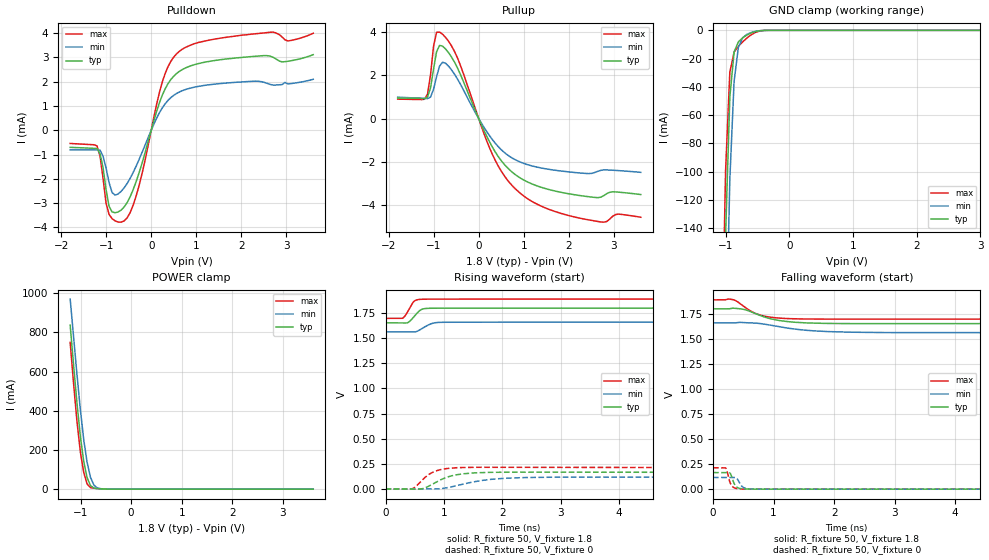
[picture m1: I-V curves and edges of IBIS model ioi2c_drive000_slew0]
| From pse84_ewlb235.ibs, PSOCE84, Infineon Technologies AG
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[Model] ioi2c_drive000_slew0
Model_type I/O
Enable   Active-High
Vinl  =  0.54
Vinh  =  1.26
Vmeas =  0.9
Cref  =  15e-12
| Capacitance   typ   min   max
C_comp   8.55364e-13 8.30808e-13 8.84570e-13
| Variables   typ   min   max
[GND Clamp Reference]   0   0   0
[POWER Clamp Reference]   1.8   1.66   1.89
[Pulldown Reference]   0   0   0
[Pullup Reference]   1.8   1.66   1.89
[Temperature Range]   25   125   -40
[Voltage Range]   1.8   1.66   1.89
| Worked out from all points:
|   slope of the pulldown table from 0 to 0.27 V, typ, clamps not added: 175 ohm
|   slope of the pullup table from 0 to 0.27 V, typ, clamps not added: 228 ohm
|   GND clamp passes 1 mA (typ) near -0.55 V on its own axis
|   POWER clamp passes 1 mA (typ) near -0.55 V on its own axis
|   falling waveform, R_fixture 50, V_fixture 1.8: 20-80 % time 476ps typ, 695ps min, 340ps max; typ from 1.8 V to 1.65 V
|   falling waveform, R_fixture 50, V_fixture 0: 20-80 % time 68.6ps typ, 76ps min, 64.6ps max; typ from 0.166 V to 0 V
|   rising waveform, R_fixture 50, V_fixture 1.8: 20-80 % time 136ps typ, 180ps min, 114ps max; typ from 1.65 V to 1.8 V
|   rising waveform, R_fixture 50, V_fixture 0: 20-80 % time 386ps typ, 627ps min, 275ps max; typ from 0 V to 0.166 V
[GND Clamp]
| Voltage   I(typ)   I(min)   I(max)
-1.204V   -750.5mA   -844.3mA   -692.2mA
-1.07V    -311.8mA   -416.8mA   -250.3mA
-1.003V   -144.6mA   -236.7mA   -99.35mA
-936.6mV  -47.15mA   -105.3mA   -29.57mA
-869.7mV  -15.32mA   -36.11mA   -15.4mA
-802.8mV  -8.178mA   -12.13mA   -11.32mA
-735.9mV  -5.345mA   -5.294mA   -8.218mA
-669mV    -3.361mA   -2.852mA   -5.471mA
-535.2mV  -838.5uA   -772.4uA   -1.486mA
-401.4mV  -47.36uA   -84.85uA   -76.78uA
3.6V      0A         0A         0A
[POWER Clamp]
| Voltage   I(typ)   I(min)   I(max)
-1.204V   837.3mA    970.7mA    749.2mA
-1.137V   634.9mA    778.2mA    540.5mA
-1.07V    440.1mA    587.4mA    346.5mA
-1.003V   270mA      407mA      190.9mA
-936.6mV  141.8mA    252.7mA    85.92mA
-869.7mV  58.74mA    136.5mA    26.66mA
-802.8mV  18.35mA    60.36mA    8.197mA
-735.9mV  5.885mA    21mA       4.755mA
-669mV    2.866mA    6.628mA    3.138mA
-334.5mV  12.31uA    45.7uA     5.857uA
3.6V      0A         0A         0A
[Pulldown]
| Voltage   I(typ)   I(min)   I(max)
-1.8V     -703.5uA   -804.7uA   -543.5uA
-1.204V   -750.4uA   -810.1uA   -642.3uA
-1.07V    -1.533mA   -1.068mA   -1.965mA
-1.003V   -2.436mA   -1.548mA   -2.997mA
-936.6mV  -3.129mA   -2.15mA    -3.46mA
-802.8mV  -3.395mA   -2.671mA   -3.729mA
-602.1mV  -3.161mA   -2.372mA   -3.733mA
-267.6mV  -1.741mA   -1.195mA   -2.266mA
248.3mV   1.454mA    928.2uA    1.997mA
558.6mV   2.33mA     1.51mA     3.138mA
1.552V    2.909mA    1.927mA    3.798mA
3.6V      3.114mA    2.1mA      3.995mA
[Pullup]
| Voltage   I(typ)   I(min)   I(max)
-1.8V     951.6uA    988.2uA    898.4uA
-1.204V   922.4uA    930.7uA    894.6uA
-1.07V    1.418mA    994.1uA    2.027mA
-1.003V   2.285mA    1.355mA    3.351mA
-936.6mV  3.088mA    1.933mA    3.984mA
-869.7mV  3.379mA    2.427mA    3.995mA
-735.9mV  3.214mA    2.556mA    3.747mA
-468.3mV  2.324mA    1.816mA    2.785mA
372.4mV   -1.557mA   -1.149mA   -1.949mA
869mV     -2.67mA    -1.957mA   -3.349mA
2.256V    -3.556mA   -2.512mA   -4.603mA
3.6V      -3.507mA   -2.482mA   -4.555mA
[Ramp]
dV/dt_r   99.4337m/0.386427n  70.1274m/0.62743n  0.128322/0.274687n
dV/dt_f   87.9626m/0.476036n  57.8568m/0.695026n  0.115304/0.339972n
R_load = 50
[Falling Waveform]
R_fixture = 50
V_fixture = 1.8
V_fixture_min = 1.66
V_fixture_max = 1.89
| Time   V(typ)   V(min)   V(max)
0s        1.8V       1.66V      1.89V
258.8ps   1.8V       1.66V      1.898V
338.3ps   1.807V     1.66V      1.89V
507.2ps   1.795V     1.663V     1.825V
666.8ps   1.761V     1.659V     1.764V
922.4ps   1.706V     1.641V     1.719V
1.326ns   1.667V     1.6V       1.701V
1.676ns   1.658V     1.58V      1.698V
2.292ns   1.653V     1.567V     1.697V
800ns     1.653V     1.564V     1.698V
[Falling Waveform]
R_fixture = 50
V_fixture = 0
V_fixture_min = 0
V_fixture_max = 0
| Time   V(typ)   V(min)   V(max)
0s        165.7mV    116.9mV    213.9mV
207.8ps   165.6mV    116.9mV    211.2mV
225.6ps   165.4mV    116.9mV    190.6mV
288.5ps   152.7mV    116.8mV    55.14mV
367.6ps   36.19mV    116.7mV    8.924mV
402ps     16.97mV    100.6mV    4.24mV
471.7ps   4.071mV    31.36mV    927.8uV
543.3ps   1.155mV    6.985mV    549.8uV
1.128ns   210.9uV    305.1uV    131.4uV
800ns     16.91nV    963.9nV    7.235nV
[Rising Waveform]
R_fixture = 50
V_fixture = 1.8
V_fixture_min = 1.66
V_fixture_max = 1.89
| Time   V(typ)   V(min)   V(max)
0s        1.653V     1.564V     1.698V
295.6ps   1.654V     1.564V     1.701V
341.2ps   1.653V     1.564V     1.728V
398.5ps   1.661V     1.564V     1.785V
476.5ps   1.707V     1.562V     1.861V
549ps     1.756V     1.572V     1.884V
641.3ps   1.792V     1.602V     1.889V
845.2ps   1.799V     1.654V     1.889V
1.344ns   1.8V       1.659V     1.89V
800ns     1.8V       1.66V      1.89V
[Rising Waveform]
R_fixture = 50
V_fixture = 0
V_fixture_min = 0
V_fixture_max = 0
| Time   V(typ)   V(min)   V(max)
0s        16.91nV    963.7nV    7.235nV
439.2ps   -1.275mV   139uV      -734.5uV
623.2ps   1.708mV    -929.8uV   85.19mV
749.9ps   30.31mV    -1.076mV   147.6mV
919.7ps   84.08mV    1.59mV     189.7mV
1.196ns   139.3mV    29.85mV    210.3mV
1.553ns   160.6mV    75.03mV    215.6mV
2.387ns   167.2mV    113.5mV    214.8mV
3.759ns   166.2mV    117.9mV    213.9mV
50ns      165.7mV    116.9mV    213.9mV
